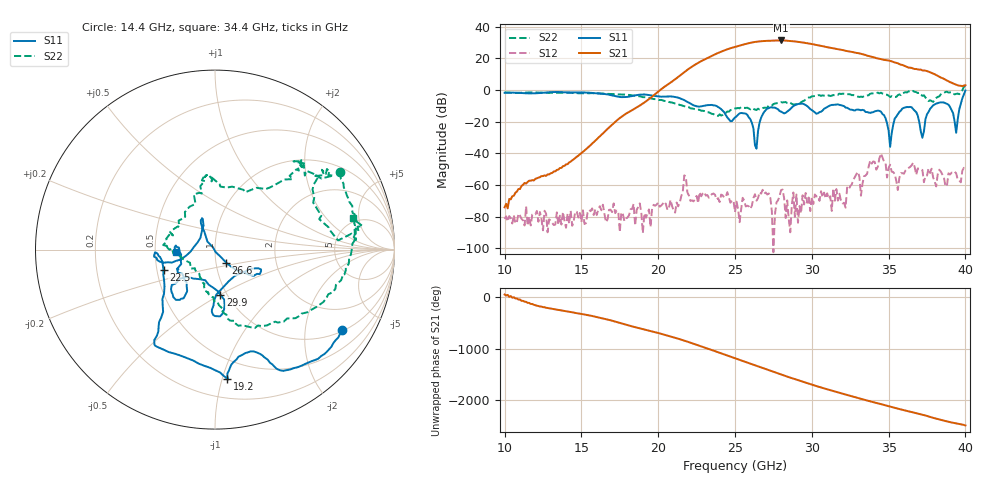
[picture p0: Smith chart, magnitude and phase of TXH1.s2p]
!Keysight Technologies,M9808A,MY58100618,A.14.70.03
!Date: Monday, February 27, 2023 13:36:43
!Correction: S11(C  2-Port  )
!S21(C  2-Port  )
!S12(C  2-Port  )
!S22(C  2-Port  )
!S2P File: Measurements: S11, S21, S12, S22:
# Hz S  RI  R 50
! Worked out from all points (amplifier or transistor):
!   301 points, 10 GHz to 40 GHz, reference 50 ohm
!   highest |S21| = 31.4 dB at 28 GHz (marker M1)
!   |S21| within 3 dB of that: 25.4 GHz to 30.38 GHz (4.98 GHz wide, 17.9 % of centre)
!   unconditionally stable (mu >= 1): start of sweep to 39.8 GHz
!   at 15 GHz: K = 76678.22, MAG = -30.1 dB, |S12| = -83.4 dB
!   at 25 GHz: K = 140.53, MAG = 27.7 dB, |S12| = -77.1 dB
!   at 40 GHz: K = -7.61, MSG = 26.7 dB, |S12| = -50.3 dB
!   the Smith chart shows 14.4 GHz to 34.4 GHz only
!   S11 on the Smith chart (normalised r, x): 14.4 GHz: 1.04, -3.12; 19.2 GHz: 0.35, -1.04; 22.5 GHz: 0.54, -0.14; 26.6 GHz: 1.12, -0.16; 29.9 GHz: 0.93, -0.50; 34.4 GHz: 0.64, -0.02
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1e10  0.7421 0.3566  0.00012 0.000158  -8.28e-05 1.87e-05  -0.0275 0.8539
1.44e10  0.7065 -0.4493  0.00238 0.00555  3.42e-05 3.84e-05  0.6954 0.4312
1.5e10  0.6367 -0.5546  0.00843 0.00575  -1.74e-06 -6.76e-05  0.7344 0.3032
1.92e10  0.0668 -0.7184  0.0286 0.4397  -8.18e-05 -4.31e-05  0.449 -0.3819
2e10  -0.1203 -0.6184  0.8118 0.3784  -0.000224 0.00017  0.2607 -0.426
2.25e10  -0.2868 -0.1143  -6.151 2.92  0.000452 -4.58e-05  -0.0412 -0.2385
2.41e10  -0.2405 -0.0723  16.13 -3.204  -0.000401 0.000302  -0.1393 -0.0731
2.5e10  -0.0701 0.1169  -6.86 -22.2  -0.00014 -3.05e-06  -0.2622 0.00762
2.58e10  -0.0783 0.1463  -28.99 5.812  0.000187 0.000122  -0.2719 0.06
2.66e10  0.0615 -0.0719  4.53 34.59  0.000427 0.00042  -0.1685 0.178
2.74e10  0.2567 -0.1188  36.59 -0.862  9.53e-05 -0.000113  -0.074 0.3121
2.8e10  0.1703 -0.1211  16.59 -33.17  -0.000393 -0.000576  -0.0456 0.4162
2.84e10  0.0521 -0.2028  -9.201 -35.09  -0.000132 0.000301  -0.016 0.3914
2.9e10  -0.0175 -0.3474  -32.76 -9.288  -0.000363 0.000348  0.0951 0.351
2.99e10  0.0294 -0.2511  -9.217 27.77  -0.000139 -5.85e-05  0.4156 0.4114
3e10  0.0165 -0.2321  -4.472 28.16  0.000226 0.000343  0.4541 0.4471
3.09e10  -0.2084 -0.1781  22.21 6.723  -0.00026 0.000274  0.4882 0.4687
3.2e10  -0.1758 -0.2715  4.235 -17.91  -0.000253 7.52e-05  0.6375 0.4362
3.3e10  -0.2078 -0.1259  -13.95 -4.939  -0.00259 0.000216  0.553 0.2896
3.44e10  -0.2198 -0.0116  0.4727 9.752  -0.00549 -0.00436  0.7665 0.1745
3.5e10  -0.0392 -0.035  6.549 5.584  0.00128 -0.00322  0.6625 0.0845
4e10  0.4704 -0.8497  1.304 0.588  -0.00303 -0.000311  1.124 -0.8778
